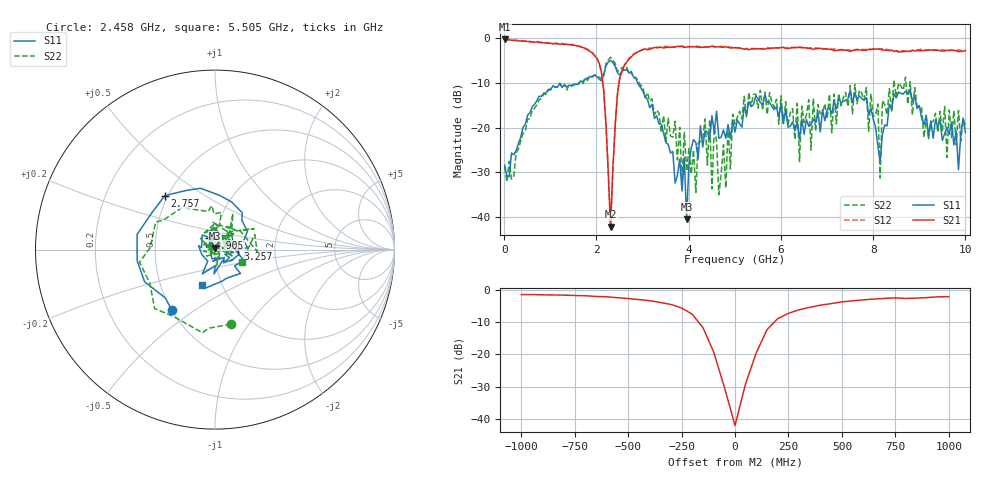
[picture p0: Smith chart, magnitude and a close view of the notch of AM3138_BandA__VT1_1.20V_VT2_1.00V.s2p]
! Date/Time: Tue, Nov 13, 2018 4:42 PM
! Network Analyzer: Agilent Technologies E8364B Rev: A.07.50.67
! Sweep from 0.010 to 10.000 GHz, 201 Points, Sweep Type: LIN
! Power Supply: 1.200 V, 0.000 A
# Hz S DB R 50
!freq MagS11 AngS11 MagS21 AngS21 MagS12 AngS12 MagS22 AngS22
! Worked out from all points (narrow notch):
!   201 points, 10 MHz to 10 GHz, reference 50 ohm
!   highest |S21| = -0.25 dB at 10 MHz (marker M1); lowest = -42.1 dB at 2.308 GHz (marker M2)
!   notch at M2: 39.7 dB deep, 171 MHz wide at half that depth
!   lowest |S11| = -40.5 dB at 3.956 GHz (marker M3), VSWR 1.02, Z = 50.2 + j0.933 ohm
!   |S11| at or under -10 dB: start of sweep to 1.627 GHz; 2.894 GHz to end of sweep
!   |S22| runs from -35.0 to -4.3 dB; largest |S21 - S12| = 0.037
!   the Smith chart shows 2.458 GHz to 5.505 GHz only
!   S11 on the Smith chart (normalised r, x): 2.458 GHz: 0.50, -0.41; 2.757 GHz: 0.48, +0.35; 3.257 GHz: 1.29, +0.01; 4.905 GHz: 0.93, +0.13; 5.505 GHz: 0.81, -0.33
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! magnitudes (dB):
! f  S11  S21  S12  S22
! 10 MHz  -28.4  -0.3  -0.2  -28.8
! 1.708 GHz  -9.7  -2.1  -2.0  -10.2
! 2.108 GHz  -9.5  -7.5  -7.5  -9.2
! 2.308 GHz  -5.0  -42.1  -42.3  -4.3
! 2.458 GHz  -7.7  -12.3  -12.4  -7.4
! 2.757 GHz  -7.7  -4.2  -4.1  -7.4
! 3.257 GHz  -17.9  -2.1  -2.2  -17.1
! 3.357 GHz  -19.2  -2.1  -2.1  -16.7
! 3.956 GHz  -40.5  -2.0  -1.9  -29.7
! 4.256 GHz  -19.6  -2.1  -1.9  -23.1
! 4.905 GHz  -22.5  -2.2  -2.1  -29.2
! 5.005 GHz  -21.0  -2.1  -2.0  -19.2
! 5.505 GHz  -13.5  -2.4  -2.3  -15.7
! 6.354 GHz  -18.7  -2.1  -2.3  -14.6
! 6.404 GHz  -22.7  -2.1  -2.0  -27.6
! 6.703 GHz  -18.1  -2.5  -2.2  -13.5
! 7.852 GHz  -13.3  -2.7  -2.5  -11.0
! 8.102 GHz  -23.9  -2.5  -2.4  -14.7
! 8.152 GHz  -27.6  -2.5  -2.4  -31.3
! 8.202 GHz  -21.4  -2.7  -2.4  -14.0
! 8.352 GHz  -14.8  -2.8  -2.8  -11.3
! 10 GHz  -21.1  -2.8  -2.7  -19.4
